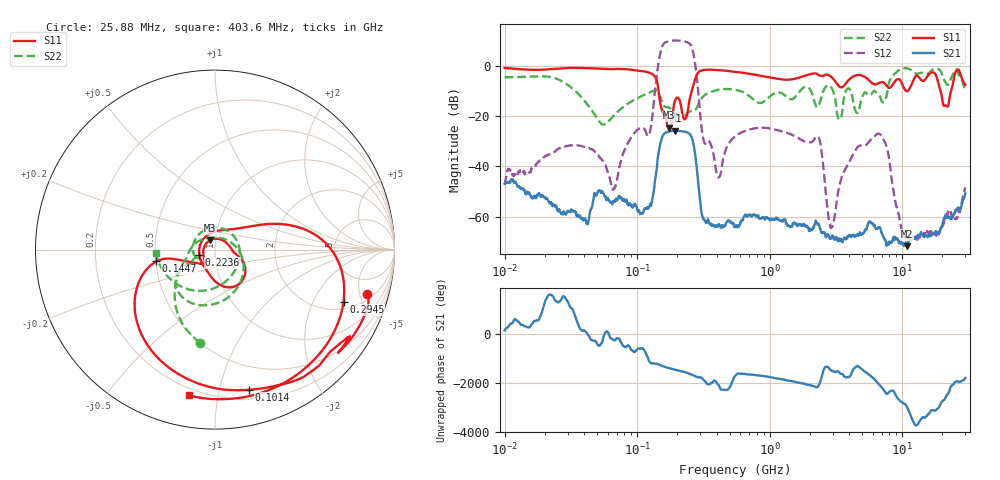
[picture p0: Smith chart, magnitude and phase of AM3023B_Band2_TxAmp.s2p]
# Hz S DB R 50.0
!freq dBS11 angS11 dBS21 angS21 dBS12 angS12 dBS22 angS22
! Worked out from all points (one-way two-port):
!   1601 points, 10 MHz to 30 GHz, reference 50 ohm
!   highest |S21| = -25.79 dB at 194.4 MHz (marker M1); lowest = -71.8 dB at 10.92 GHz (marker M2)
!   lowest |S11| = -24.6 dB at 175 MHz (marker M3), VSWR 1.13, Z = 47 + j4.88 ohm
!   |S11| at or under -10 dB: 145 MHz to 258.3 MHz (113.3 MHz wide, 56.2 % of centre); 10.72 GHz to 11.03 GHz (311.2 MHz wide, 2.86 % of centre); 19.49 GHz to 23.39 GHz (3.903 GHz wide, 18.2 % of centre)
!   |S22| runs from -23.4 to -0.9 dB; largest |S21 - S12| = 3.2
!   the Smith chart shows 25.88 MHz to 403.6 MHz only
!   S11 on the Smith chart (normalised r, x): 25.88 MHz: 2.64, -5.92; 101.4 MHz: 0.28, -1.23; 144.7 MHz: 0.50, -0.07; 223.6 MHz: 0.84, -0.05; 294.5 MHz: 2.43, -3.52; 403.6 MHz: 0.16, -0.82
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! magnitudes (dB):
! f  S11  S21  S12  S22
! 10 MHz  -0.8  -47.0  -47.2  -4.5
! 25.88 MHz  -1.1  -57.1  -32.9  -5.6
! 38.04 MHz  -0.9  -60.9  -31.9  -12.5
! 66.63 MHz  -1.3  -53.8  -49.1  -19.8
! 101.4 MHz  -1.9  -57.9  -25.3  -12.8
! 123.9 MHz  -2.8  -55.8  -27.0  -10.6
! 144.7 MHz  -9.5  -35.1  0.8  -10.5
! 175 MHz  -24.6  -26.1  9.8  -16.6
! 194.4 MHz  -13.5  -25.8  10.1  -19.2
! 223.6 MHz  -20.7  -26.1  9.8  -19.9
! 262.5 MHz  -8.7  -29.7  6.1  -18.2
! 294.5 MHz  -2.2  -50.7  -15.0  -14.4
! 403.6 MHz  -1.7  -63.8  -43.8  -9.6
! 547.7 MHz  -2.4  -64.2  -28.1  -9.5
! 2.084 GHz  -3.2  -65.5  -30.3  -10.9
! 2.397 GHz  -3.9  -64.8  -30.1  -14.6
! 2.928 GHz  -4.5  -68.6  -64.2  -8.7
! 3.352 GHz  -8.2  -68.7  -47.9  -21.4
! 4.571 GHz  -3.7  -67.2  -32.6  -18.8
! 7.926 GHz  -8.8  -70.8  -36.2  -7.0
! 10.92 GHz  -10.1  -71.8  -68.6  -1.0
! 30 GHz  -7.6  -50.7  -48.4  -9.3
